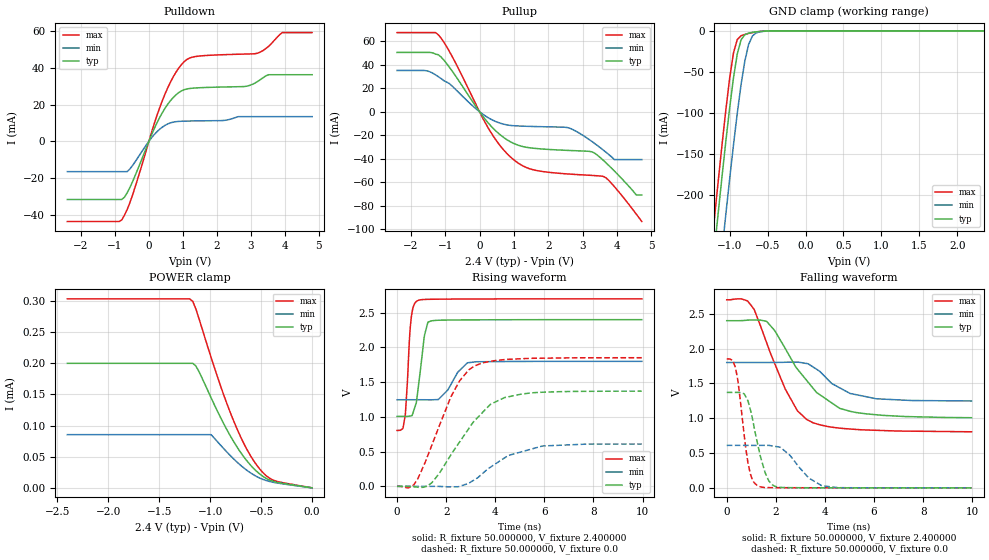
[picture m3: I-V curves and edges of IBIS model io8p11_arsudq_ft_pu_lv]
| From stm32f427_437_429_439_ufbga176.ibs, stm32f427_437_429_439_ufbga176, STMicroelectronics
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|   Model io8p11_arsudq_ft_pu_lv
[Model]  io8p11_arsudq_ft_pu_lv
Model_type I/O
Polarity   Non-Inverting
Enable   Active-Low
Vinl =   0.720000V
Vinh =   1.680000V
Vmeas =  1.200000V
Cref =   30.000000pF
Rref =   100.000000M
Vref =   0.0V
C_comp   2.239000pF   2.178700pF   2.334000pF
[Temperature Range]   25.000000   0.125000k   -40.000000
[Pullup Reference]   2.400000V   1.800000V   2.700000V
[Pulldown Reference]   0.0V   0.0V   0.0V
[POWER Clamp Reference]   2.400000V   1.800000V   2.700000V
[GND Clamp Reference]   0.0V   0.0V   0.0V
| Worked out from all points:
|   slope of the pulldown table from 0 to 0.36 V, typ, clamps not added: 25 ohm
|   slope of the pullup table from 0 to 0.36 V, typ, clamps not added: 27.7 ohm
|   GND clamp passes 1 mA (typ) near -0.62 V on its own axis
|   rising waveform, R_fixture 50.000000, V_fixture 2.400000: 20-80 % time 281ps typ, 622ps min, 183ps max; typ from 1.01 V to 2.4 V
|   rising waveform, R_fixture 50.000000, V_fixture 0.0: 20-80 % time 1.69ns typ, 1.69ns min, 1.31ns max; typ from 0.001 V to 1.37 V
|   falling waveform, R_fixture 50.000000, V_fixture 2.400000: 20-80 % time 1.82ns typ, 1.3ns min, 1.38ns max; typ from 2.4 V to 1.01 V
|   falling waveform, R_fixture 50.000000, V_fixture 0.0: 20-80 % time 536ps typ, 926ps min, 384ps max; typ from 1.37 V to 0.001 V
[Pulldown]
|Voltage   I(typ)   I(min)   I(max)
-2.4V     -31.73mA   -16.51mA   -43.74mA
-800mV    -31.73mA   -16.51mA   -42.87mA
-480mV    -21.98mA   -13.17mA   -29.21mA
80mV      3.63mA     1.966mA    5.014mA
480mV     18.16mA    8.738mA    26.02mA
800mV     25.38mA    10.72mA    37.77mA
1.12V     28.53mA    11.02mA    44.6mA
2.8V      29.84mA    13.46mA    47.53mA
3.2V      32.6mA     13.46mA    48.03mA
3.52V     36.28mA    13.46mA    51.75mA
3.92V     36.28mA    13.46mA    59.24mA
4.8V      36.28mA    13.46mA    59.24mA
[Pullup]
|Voltage   I(typ)   I(min)   I(max)
-2.4V     50.44mA    35.08mA    67.32mA
-1.52V    50.44mA    34.74mA    67.32mA
-1.2V     48.5mA     29.88mA    65.48mA
320mV     -11.75mA   -6.207mA   -17.08mA
1.04V     -27.53mA   -11.97mA   -41.91mA
1.6V      -31.13mA   -12.57mA   -49.63mA
2.56V     -32.88mA   -13.48mA   -52.9mA
3.28V     -34.18mA   -25.52mA   -54.17mA
3.6V      -41.3mA    -32.62mA   -54.97mA
3.92V     -50.32mA   -40.7mA    -63.62mA
4.56V     -70.8mA    -40.7mA    -87.07mA
4.72V     -70.8mA    -40.7mA    -93.4mA
[GND_clamp]
|Voltage   I(typ)   I(min)   I(max)
-2.4V     -1.424A    -1.508A    -1.393A
-1.25V    -311.2mA   -401.9mA   -273.3mA
-1.2V     -265.4mA   -356.1mA   -227.2mA
-1.15V    -220.4mA   -310.8mA   -181.9mA
-1.1V     -176.3mA   -266.2mA   -137.9mA
-1.05V    -133.8mA   -222.5mA   -95.87mA
-950mV    -57.3mA    -138.9mA   -26.98mA
-900mV    -28.27mA   -100.4mA   -10.59mA
-850mV    -11.01mA   -65.54mA   -5.958mA
-750mV    -2.834mA   -16.5mA    -3.178mA
-600mV    -750uA     -1.164mA   -738.3uA
2.35V     0A         0A         0A
[POWER_clamp]
|Voltage   I(typ)   I(min)   I(max)
-2.4V     200uA      85.39uA    303.5uA
-1.2V     200uA      85.39uA    303.5uA
-1.17V    200uA      85.39uA    299.5uA
-1.14V    195.7uA    85.39uA    287.5uA
-990mV    144.6uA    85.39uA    209.3uA
-870mV    104.1uA    63.61uA    150.8uA
-780mV    77.28uA    48.2uA     111.8uA
-660mV    47.71uA    30.75uA    68.21uA
-570mV    30.64uA    20.61uA    42.79uA
-480mV    18.19uA    13.44uA    24.07uA
-390mV    10.91uA    9.231uA    13.01uA
0V        0A         0A         0A
[Ramp]
| variable   typ   min   max
dV/dt_r  0.82177/1.69243n   0.36422/1.68167n   1.11101/1.31438n
dV/dt_f  0.83184/1.81553n   0.33240/1.30060n   1.13516/1.37416n
R_load = 50.000000
[Rising Waveform]
R_fixture= 50.000000
V_fixture= 2.400000
V_fixture_min= 1.800000
V_fixture_max= 2.700000
|time   V(typ)   V(min)   V(max)
0s        1.007V     1.247V     805.7mV
240.2ps   1.007V     1.247V     833.3mV
340.3ps   1.007V     1.247V     1.039V
500.5ps   1.012V     1.247V     2.084V
580.6ps   1.016V     1.247V     2.432V
840.8ps   1.354V     1.247V     2.674V
1.121ns   2.178V     1.247V     2.691V
1.361ns   2.379V     1.246V     2.693V
2.883ns   2.397V     1.78V      2.697V
9.97ns    2.4V       1.8V       2.699V
[Rising Waveform]
R_fixture= 50.000000
V_fixture= 0.0
V_fixture_min= 0.0
V_fixture_max= 0.0
|time   V(typ)   V(min)   V(max)
0s        1.05mV     906.1uV    1.468mV
680.7ps   -4.519mV   891.9uV    23.49mV
1.421ns   54.09mV    940.8uV    596.9mV
2.202ns   457.4mV    -5.839mV   1.294V
2.543ns   636.4mV    628.3uV    1.516V
3.143ns   939.5mV    93.37mV    1.73V
3.804ns   1.182V     276.1mV    1.8V
4.364ns   1.276V     406.7mV    1.825V
5.926ns   1.355V     581.5mV    1.846V
9.97ns    1.371V     610.1mV    1.852V
[Falling Waveform]
R_fixture= 50.000000
V_fixture= 2.400000
V_fixture_min= 1.800000
V_fixture_max= 2.700000
|time   V(typ)   V(min)   V(max)
0s        2.4V       1.8V       2.699V
620.6ps   2.401V     1.8V       2.711V
1.101ns   2.41V      1.8V       2.569V
1.622ns   2.391V     1.8V       2.087V
2.382ns   2.002V     1.803V     1.42V
2.883ns   1.704V     1.805V     1.105V
3.263ns   1.54V      1.785V     981mV
3.664ns   1.368V     1.702V     918.9mV
5.065ns   1.097V     1.353V     844.5mV
9.97ns    1.007V     1.247V     805.7mV
[Falling Waveform]
R_fixture= 50.000000
V_fixture= 0.0
V_fixture_min= 0.0
V_fixture_max= 0.0
|time   V(typ)   V(min)   V(max)
0s        1.371V     610.1mV    1.852V
360.4ps   1.371V     610.2mV    1.719V
460.5ps   1.37V      610.1mV    1.523V
720.7ps   1.345V     610.1mV    730.1mV
961ps     1.125V     609.9mV    202mV
1.281ns   594.9mV    609.8mV    27.87mV
1.702ns   109.4mV    610.9mV    4.556mV
2.062ns   13.71mV    591.1mV    3.226mV
3.884ns   1.919mV    30.9mV     2.052mV
9.97ns    1.05mV     906.1uV    1.468mV
